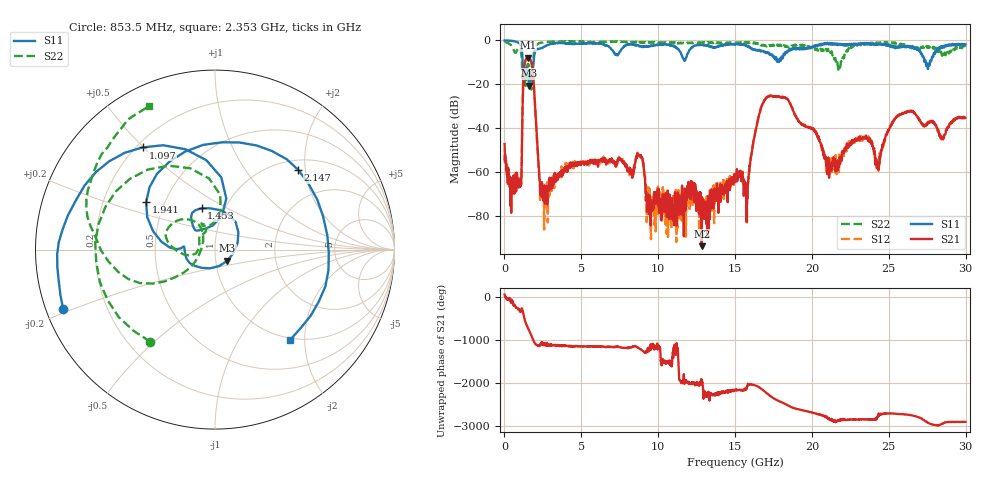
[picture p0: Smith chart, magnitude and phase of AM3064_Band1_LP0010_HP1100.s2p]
# Hz S DB R 50.0
!freq dBS11 angS11 dBS21 angS21 dBS12 angS12 dBS22 angS22
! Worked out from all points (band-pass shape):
!   1600 points, 10 MHz to 29.98 GHz, reference 50 ohm
!   highest |S21| = -7.97 dB at 1.528 GHz (marker M1); lowest = -94.0 dB at 12.83 GHz (marker M2)
!   |S21| within 3 dB of the highest: 1.307 GHz to 1.781 GHz (473.9 MHz wide, 30.7 % of centre)
!   lowest |S11| = -20.6 dB at 1.603 GHz (marker M3), VSWR 1.20, Z = 56.9 - j7.16 ohm
!   |S11| at or under -10 dB: 1.186 GHz to 1.889 GHz (703.2 MHz wide, 45.7 % of centre); 27.4 GHz to 27.68 GHz (281.9 MHz wide, 1.02 % of centre)
!   |S22| runs from -22.5 to -0.3 dB; largest |S21 - S12| = 0.0067
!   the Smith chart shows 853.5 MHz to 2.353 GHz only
!   S11 on the Smith chart (normalised r, x): 853.5 MHz: 0.05, -0.19; 1.097 GHz: 0.22, +0.50; 1.453 GHz: 0.78, +0.38; 1.941 GHz: 0.39, +0.27; 2.147 GHz: 1.21, +1.83; 2.353 GHz: 0.96, -1.69
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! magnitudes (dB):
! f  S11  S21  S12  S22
! 10 MHz  -0.1  -47.3  -52.5  -0.3
! 853.5 MHz  -0.8  -64.4  -63.9  -4.1
! 1.097 GHz  -3.1  -63.2  -63.8  -6.5
! 1.453 GHz  -12.3  -8.2  -8.1  -13.5
! 1.528 GHz  -14.4  -8.0  -7.9  -10.7
! 1.603 GHz  -20.6  -8.1  -8.1  -11.9
! 1.941 GHz  -6.6  -23.8  -23.7  -5.1
! 2.147 GHz  -3.8  -48.8  -48.7  -1.8
! 2.353 GHz  -3.7  -70.7  -69.8  -1.1
! 5.015 GHz  -1.4  -55.6  -55.3  -0.7
! 8.801 GHz  -2.6  -52.9  -52.5  -0.9
! 10 GHz  -2.0  -75.5  -74.2  -0.9
! 12.83 GHz  -2.1  -94.0  -79.4  -1.0
! 15 GHz  -1.8  -64.6  -62.9  -1.2
! 15.75 GHz  -2.4  -83.0  -71.4  -0.8
! 17.14 GHz  -5.9  -25.7  -25.6  -2.7
! 19.99 GHz  -3.4  -40.4  -40.2  -3.4
! 21.12 GHz  -1.3  -62.8  -61.6  -5.0
! 23.36 GHz  -1.6  -44.0  -45.0  -1.9
! 24.25 GHz  -1.7  -58.5  -58.1  -1.5
! 25 GHz  -2.0  -41.1  -41.0  -1.2
! 29.98 GHz  -1.9  -35.4  -35.2  -3.1
